(* 	
	Program Name: 	ACS_CMD_STOP_MOTION
	Purpose:		Copy Stop Motion Command to ACS Drive Output Command Register
	When Executed:	Stops current motion profile at defined profile deceleration
*)
PROGRAM ACS_CMD_STOP_MOTION
VAR_IN_OUT
	Axis:ACS_DRIVE_TYPE;
END_VAR
VAR
	_command:	USINT	:= ACS_COMMANDS.STOP_MOTION;
END_VAR

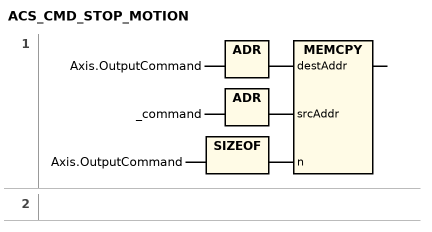
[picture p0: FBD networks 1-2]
// NETWORK 1
MEMCPY(destAddr := ADR(Axis.OutputCommand), srcAddr := ADR(_command), n := SIZEOF(Axis.OutputCommand));

// NETWORK 2

END_PROGRAM
